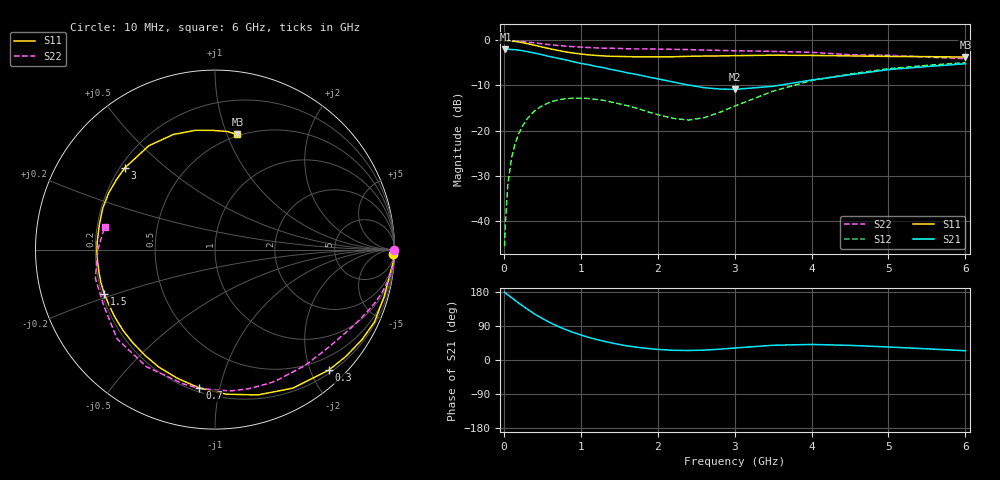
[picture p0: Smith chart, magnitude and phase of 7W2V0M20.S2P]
! Infineon Technologies  Discrete & RF Semiconductors
! BFS17W
! Si NPN RF Bipolar Junction Transistor in SOT323
! VCE = 2 V  IC = 0.2 mA
! Common Emitter S-Parameters:  August  1999
# GHz  S  MA  R  50
!  f  S11  S21  S12  S22
! GHz  MAG  ANG  MAG  ANG  MAG  ANG  MAG  ANG
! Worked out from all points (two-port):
!   36 points, 10 MHz to 6 GHz, reference 50 ohm
!   highest |S21| = -1.93 dB at 20 MHz (marker M1); lowest = -10.9 dB at 3 GHz (marker M2)
!   |S21| within 3 dB of the highest: start of sweep to 955.2 MHz
!   lowest |S11| = -3.7 dB at 6 GHz (marker M3), VSWR 4.77, Z = 24.3 + j54.5 ohm
!   |S11| at or under -10 dB: nowhere
!   |S22| runs from -4.0 to 0.0 dB; largest |S21 - S12| = 0.8
!   S11 on the Smith chart (normalised r, x): 10 MHz: 26, -66; 300 MHz: 0.25, -2.29; 700 MHz: 0.22, -0.87; 1.5 GHz: 0.21, -0.19; 3 GHz: 0.22, +0.37; 6 GHz: 0.49, +1.09
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0.01  0.9897 -1.5  0.798 179.3  0.0052 86.9  0.9999 0.0
0.02  0.9975 -3.5  0.801 177.0  0.0095 89.2  0.995 -1.0
0.05  0.9846 -8.0  0.801 172.2  0.0243 86.0  0.9982 -2.5
0.1  0.9779 -15.7  0.792 164.7  0.0496 79.5  0.9956 -5.1
0.15  0.9756 -24.5  0.789 156.7  0.073 74.1  0.9881 -7.5
0.2  0.96 -31.6  0.779 149.2  0.0948 69.8  0.9801 -9.8
0.3  0.9233 -46.7  0.754 134.9  0.1337 60.4  0.9614 -14.3
0.4  0.8856 -60.6  0.724 121.3  0.1658 51.7  0.9394 -18.4
0.5  0.8445 -73.5  0.694 109.6  0.1889 44.2  0.917 -22.0
0.7  0.7763 -96.4  0.635 89.1  0.2184 32.2  0.8807 -28.7
0.9  0.7263 -115.3  0.581 72.8  0.2282 22.7  0.8522 -34.8
1.1  0.6919 -131.7  0.538 59.7  0.2268 15.7  0.8344 -40.8
1.5  0.6644 -158.1  0.458 41.0  0.1983 7.4  0.8153 -53.1
2.2  0.6593 167.8  0.346 25.6  0.1365 19.1  0.7974 -76.4
2.6  0.6713 152.0  0.299 26.0  0.1386 42.1  0.7829 -90.2
3  0.6779 137.9  0.286 31.7  0.1867 56.8  0.769 -103.4
3.5  0.6862 122.5  0.31 38.9  0.2736 59.4  0.7559 -120.4
4  0.6822 109.9  0.364 41.0  0.3589 54.0  0.7381 -137.7
4.5  0.6736 99.3  0.416 38.6  0.4236 46.9  0.6939 -153.4
5  0.6645 91.2  0.475 34.3  0.4862 40.0  0.6854 -166.5
5.5  0.6614 84.2  0.513 29.5  0.5288 33.3  0.653 -179.9
6  0.6535 79.0  0.551 24.4  0.5674 27.2  0.6281 168.4
